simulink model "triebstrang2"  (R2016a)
settings: Solver=ode5  StartTime=0.0  StopTime=25  FixedStep=0.001  RelTol=1e-3
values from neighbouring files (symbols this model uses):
  b = zeros(N, 1)    [fourierrechteck.m]    (also in init_lorenzC.m = 28; init_pendelStange.m = 0.2)
  c = 8/3    (= 2.66666666667)    [init_lorenzC.m]
  m = 1.0    (= 1)    [init_pendelStange.m]
undefined symbols (not defined in the file or in its folder): i, J, Mg, v0, w0
libraries: simulink x1

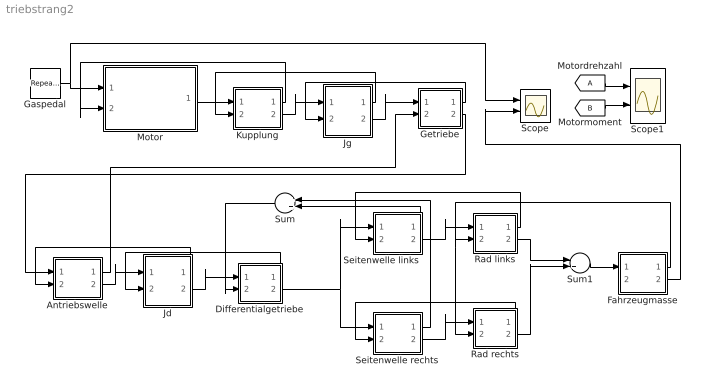
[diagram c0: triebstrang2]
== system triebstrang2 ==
  Antriebswelle : Subsystem
  Differentialgetriebe : Subsystem
  Fahrzeugmasse : Subsystem
  Gaspedal : simulink/Sources/Repeating Sequence  rep_seq_t=[0 4 4.001 8 8.001 12 12.001 16 16.001 30]  rep_seq_y=[0 0 0.3 0.3 0.6 0.6 1 1 0 0]
  Getriebe : Subsystem
  Jd : Subsystem
  Jg : Subsystem
  Kupplung : Subsystem
  Motor : Subsystem
  Motordrehzahl : From  TagVisibility=global
  Rad links : Subsystem
  Rad rechts : Subsystem
  Scope : Scope  NumInputPorts=2
  Scope1 : Scope  NumInputPorts=2
  Seitenwelle links : Subsystem
  Seitenwelle rechts : Subsystem
  Sum : Sum
  Sum1 : Sum
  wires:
  Gaspedal/1 -> Motor/1(Fahrpedalweg pf), Scope/1
  Motor/1(wr) -> Kupplung/1(wl)
  Kupplung/2(Mr) -> Jg/1(Ml)
  Jg/2(wr) -> Getriebe/1(wl)
  Kupplung/1(Ml) -> Motor/2(Mr)
  Jg/1(wl) -> Kupplung/2(wr)
  Getriebe/1(Ml) -> Jg/2(Mr)
  Antriebswelle/1(Ml) -> Getriebe/2(Mr)
  Jd/1(wl) -> Antriebswelle/2(wr)
  Jd/2(wr) -> Differentialgetriebe/1(wl)
  Differentialgetriebe/1(Ml) -> Jd/2(Mr)
  Seitenwelle links/1(Ml) -> Sum/2
  Seitenwelle rechts/1(Ml) -> Sum/1
  Sum/1 -> Differentialgetriebe/2(Mr)
  Seitenwelle links/2(Mr) -> Rad links/1(Ml)
  Seitenwelle rechts/2(Mr) -> Rad rechts/1(Ml)
  Rad links/1(wl) -> Seitenwelle links/2(wr)
  Rad rechts/1(wl) -> Seitenwelle rechts/2(wr)
  Rad links/2(Mr) -> Sum1/1
  Rad rechts/2(Mr) -> Sum1/2
  Sum1/1 -> Fahrzeugmasse/1(Fl)
  Fahrzeugmasse/1(vl) -> Rad rechts/2(wr), Rad links/2(wr)
  Fahrzeugmasse/2(vr) -> Scope/2
  Motordrehzahl/1 -> Scope1/1
  [B] -> Scope1/2
  Antriebswelle/2(Mr) -> Jd/1(Ml)
  Getriebe/2(wr) -> Antriebswelle/1(wl)
  Differentialgetriebe/2(wr) -> Seitenwelle links/1(wl), Seitenwelle rechts/1(wl)

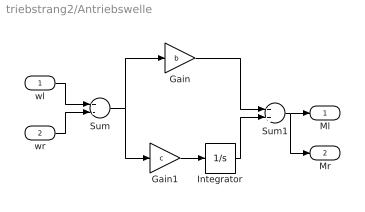
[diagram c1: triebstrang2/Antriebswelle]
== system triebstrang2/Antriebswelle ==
  wl : Inport
  wr : Inport  Port=2
  Gain : Gain  Gain=b
  Gain1 : Gain  Gain=c
  Integrator : Integrator
  Sum : Sum  Inputs=+-
  Sum1 : Sum
  Ml : Outport
  Mr : Outport  Port=2
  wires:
  Gain1/1 -> Integrator/1
  Sum/1 -> Gain1/1, Gain/1
  wr/1 -> Sum/2
  wl/1 -> Sum/1
  Integrator/1 -> Sum1/2
  Gain/1 -> Sum1/1
  Sum1/1 -> Mr/1, Ml/1

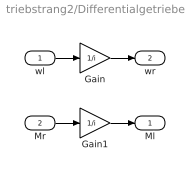
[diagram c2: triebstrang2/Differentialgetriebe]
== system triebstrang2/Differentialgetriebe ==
  wl : Inport
  Mr : Inport  Port=2
  Gain : Gain  Gain=1/i
  Gain1 : Gain  Gain=1/i
  Ml : Outport
  wr : Outport  Port=2
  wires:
  wl/1 -> Gain/1
  Gain/1 -> wr/1
  Mr/1 -> Gain1/1
  Gain1/1 -> Ml/1

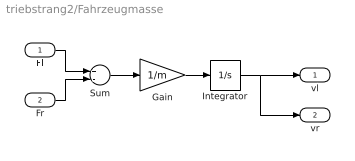
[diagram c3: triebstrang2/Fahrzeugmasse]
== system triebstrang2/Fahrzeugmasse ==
  Fl : Inport
  Fr : Inport  Port=2
  Gain : Gain  Gain=1/m
  Integrator : Integrator  InitialCondition=v0
  Sum : Sum  Inputs=+-
  vl : Outport
  vr : Outport  Port=2
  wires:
  Fl/1 -> Sum/1
  Fr/1 -> Sum/2
  Sum/1 -> Gain/1
  Gain/1 -> Integrator/1
  Integrator/1 -> vr/1, vl/1

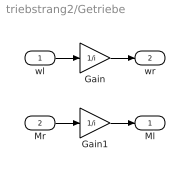
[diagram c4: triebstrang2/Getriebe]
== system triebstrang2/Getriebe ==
  wl : Inport
  Mr : Inport  Port=2
  Gain : Gain  Gain=1/i
  Gain1 : Gain  Gain=1/i
  Ml : Outport
  wr : Outport  Port=2
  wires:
  Gain1/1 -> Ml/1
  Mr/1 -> Gain1/1
  Gain/1 -> wr/1
  wl/1 -> Gain/1

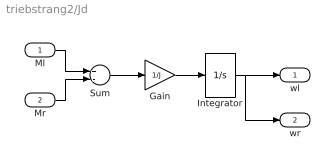
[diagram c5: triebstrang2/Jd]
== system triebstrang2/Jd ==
  Ml : Inport
  Mr : Inport  Port=2
  Gain : Gain  Gain=1/J
  Integrator : Integrator  InitialCondition=w0
  Sum : Sum  Inputs=+-
  wl : Outport
  wr : Outport  Port=2
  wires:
  Integrator/1 -> wl/1, wr/1
  Gain/1 -> Integrator/1
  Sum/1 -> Gain/1
  Mr/1 -> Sum/2
  Ml/1 -> Sum/1

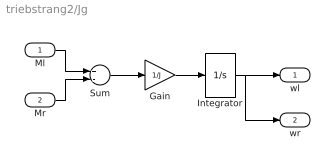
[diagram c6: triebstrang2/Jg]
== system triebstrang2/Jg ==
  Ml : Inport
  Mr : Inport  Port=2
  Gain : Gain  Gain=1/J
  Integrator : Integrator  InitialCondition=w0
  Sum : Sum  Inputs=+-
  wl : Outport
  wr : Outport  Port=2
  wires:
  Ml/1 -> Sum/1
  Mr/1 -> Sum/2
  Sum/1 -> Gain/1
  Gain/1 -> Integrator/1
  Integrator/1 -> wr/1, wl/1

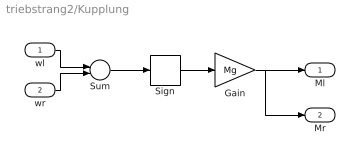
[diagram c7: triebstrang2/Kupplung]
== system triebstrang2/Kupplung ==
  wl : Inport
  wr : Inport  Port=2
  Gain : Gain  Gain=Mg
  Sign : Signum
  Sum : Sum  Inputs=+-
  Ml : Outport
  Mr : Outport  Port=2
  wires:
  wr/1 -> Sum/2
  wl/1 -> Sum/1
  Sum/1 -> Sign/1
  Sign/1 -> Gain/1
  Gain/1 -> Ml/1, Mr/1

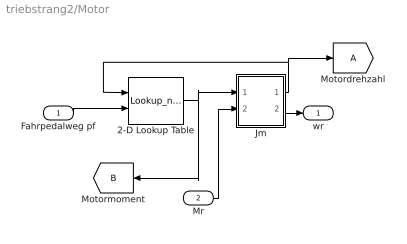
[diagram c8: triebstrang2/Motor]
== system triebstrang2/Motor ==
  Fahrpedalweg pf : Inport
  Mr : Inport  Port=2
  2-D Lookup Table : Lookup_n-D  BreakpointsForDimension1=[0:7000*pi/420:7000*pi/30]  BreakpointsForDimension2=[0:0.25:1]  Table="[-10 -10 -10 -10 -10; 22 174 186 187 188; -8 59 197 210 212; -29 24 200 217 222; -31 4 206 230 235; -40 -7 196 237 246; -44 -11 180 239 248; -46 -17 161 242 250; -59 -20 147 251 260; -72 -28 132 250 258; -76 -30 108 246 250;  -83 -32 102 222 229; -85 -42 100 200 206; -86 -62 95 180 180; -87 -87 -87 -87 -87]"  RndMeth=Simplest
  Jm : Subsystem
  Motordrehzahl : Goto  TagVisibility=global
  wr : Outport
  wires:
  Fahrpedalweg pf/1 -> 2-D Lookup Table/2
  Jm/1(wl) -> Motordrehzahl/1, 2-D Lookup Table/1
  Mr/1 -> Jm/2(Mr)
  Jm/2(wr) -> wr/1
  2-D Lookup Table/1 -> Jm/1(Ml), [B]

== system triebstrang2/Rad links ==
  Ml : Inport
  wr : Inport  Port=2
  Gain : Gain  Gain=1/i
  Gain1 : Gain  Gain=1/i
  wl : Outport
  Mr : Outport  Port=2
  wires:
  Gain1/1 -> Mr/1
  Ml/1 -> Gain1/1
  Gain/1 -> wl/1
  wr/1 -> Gain/1

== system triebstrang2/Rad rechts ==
  Ml : Inport
  wr : Inport  Port=2
  Gain : Gain  Gain=1/i
  Gain1 : Gain  Gain=1/i
  wl : Outport
  Mr : Outport  Port=2
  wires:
  wr/1 -> Gain/1
  Gain/1 -> wl/1
  Ml/1 -> Gain1/1
  Gain1/1 -> Mr/1

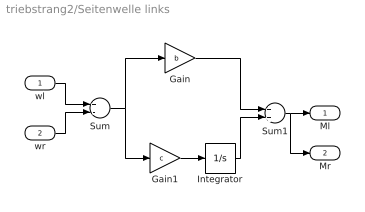
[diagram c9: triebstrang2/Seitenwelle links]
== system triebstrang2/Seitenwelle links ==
  wl : Inport
  wr : Inport  Port=2
  Gain : Gain  Gain=b
  Gain1 : Gain  Gain=c
  Integrator : Integrator
  Sum : Sum  Inputs=+-
  Sum1 : Sum
  Ml : Outport
  Mr : Outport  Port=2
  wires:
  Sum1/1 -> Ml/1, Mr/1
  Gain/1 -> Sum1/1
  Integrator/1 -> Sum1/2
  wl/1 -> Sum/1
  wr/1 -> Sum/2
  Sum/1 -> Gain/1, Gain1/1
  Gain1/1 -> Integrator/1

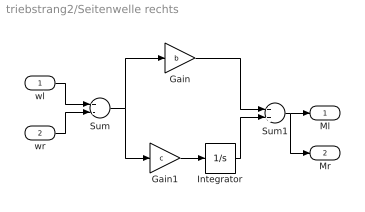
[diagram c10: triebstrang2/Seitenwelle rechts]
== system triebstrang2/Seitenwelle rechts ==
  wl : Inport
  wr : Inport  Port=2
  Gain : Gain  Gain=b
  Gain1 : Gain  Gain=c
  Integrator : Integrator
  Sum : Sum  Inputs=+-
  Sum1 : Sum
  Ml : Outport
  Mr : Outport  Port=2
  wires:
  Gain1/1 -> Integrator/1
  Sum/1 -> Gain1/1, Gain/1
  wr/1 -> Sum/2
  wl/1 -> Sum/1
  Integrator/1 -> Sum1/2
  Gain/1 -> Sum1/1
  Sum1/1 -> Mr/1, Ml/1

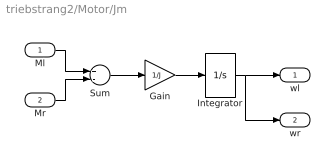
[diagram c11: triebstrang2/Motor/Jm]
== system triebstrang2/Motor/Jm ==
  Ml : Inport
  Mr : Inport  Port=2
  Gain : Gain  Gain=1/J
  Integrator : Integrator  InitialCondition=w0
  Sum : Sum  Inputs=+-
  wl : Outport
  wr : Outport  Port=2
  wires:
  Integrator/1 -> wl/1, wr/1
  Gain/1 -> Integrator/1
  Sum/1 -> Gain/1
  Mr/1 -> Sum/2
  Ml/1 -> Sum/1
